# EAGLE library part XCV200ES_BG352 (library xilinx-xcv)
xcv200es_bg352 edit this description Auto generated by make-symbol-device-package-bsdl.ulp Rev. 26 Source: xcv200es_bg352.bsd
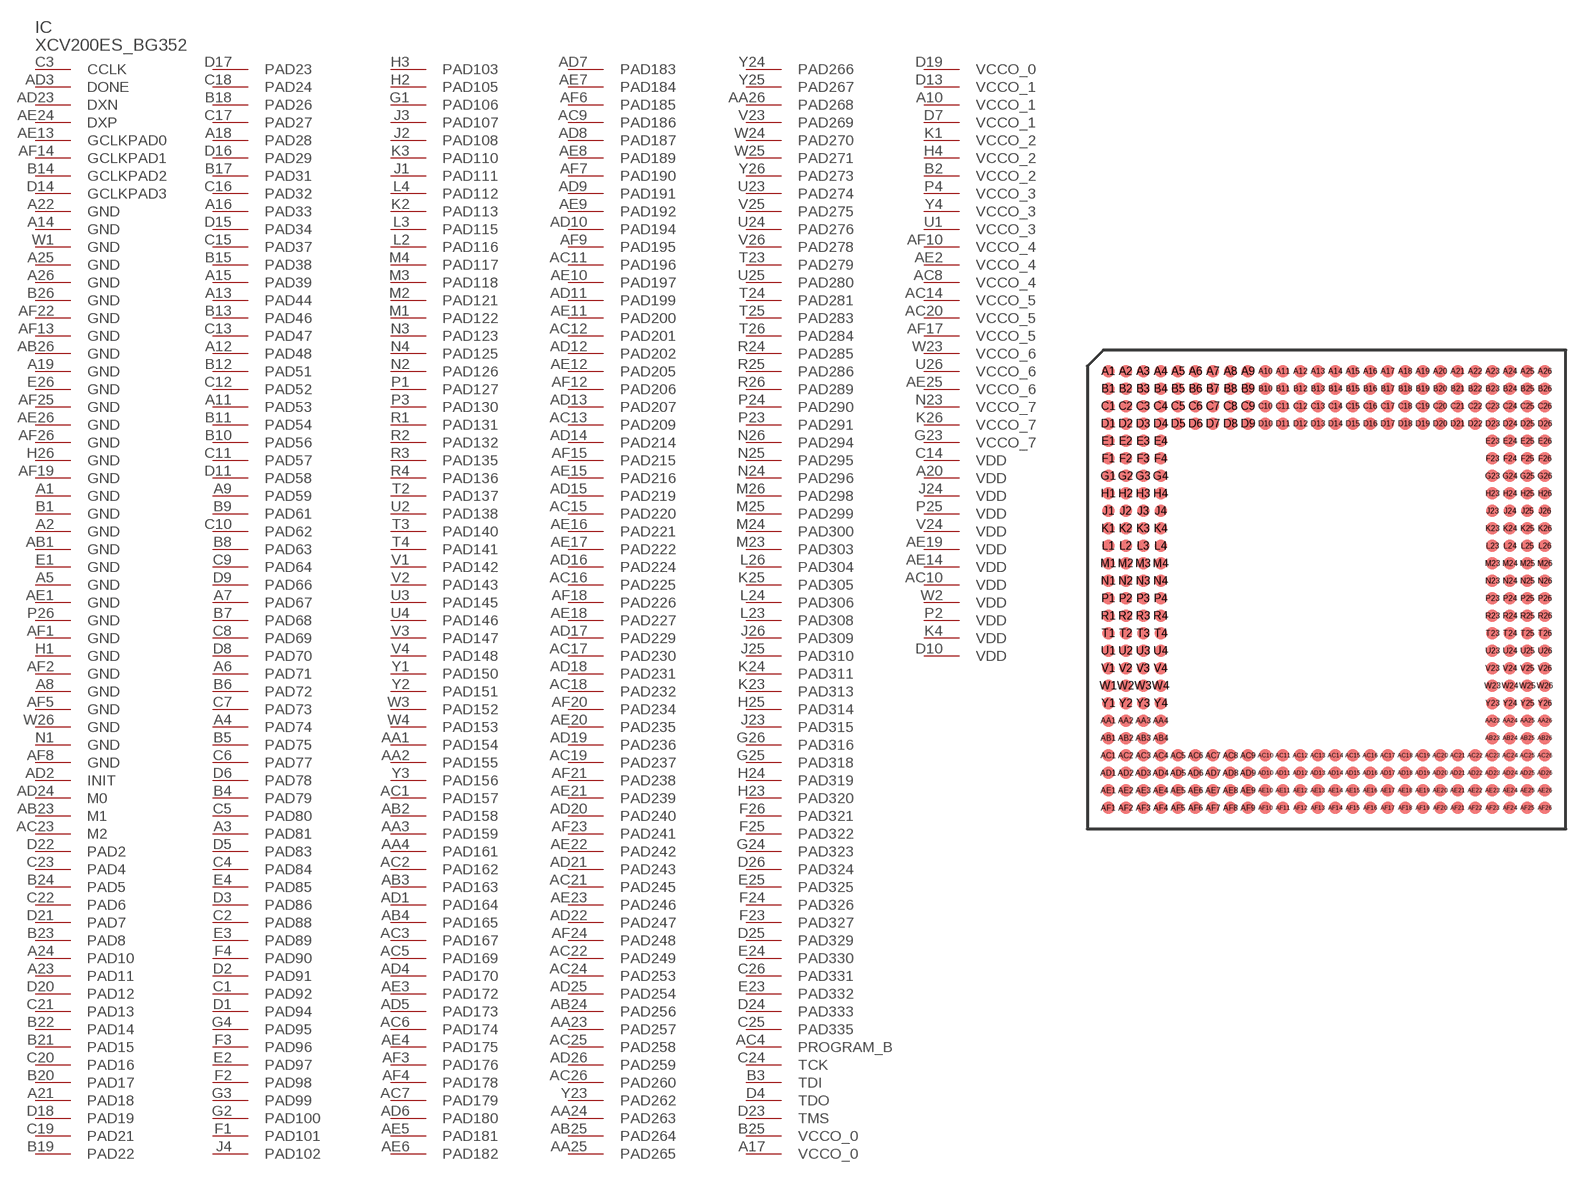
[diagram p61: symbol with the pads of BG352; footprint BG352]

Designator prefix IC

## XCV200ES_BG352 (OC_FARNELL: unknown; OC_NEWARK: unknown)  [BG352]
A1  GND  pwr
A2  GND  pwr
A3  PAD81
A4  PAD74
A5  GND  pwr
A6  PAD71
A7  PAD67
A8  GND  pwr
A9  PAD59
A10  VCCO_1  pwr
A11  PAD53
A12  PAD48
A13  PAD44
A14  GND  pwr
A15  PAD39
A16  PAD33
A17  VCCO_0  pwr
A18  PAD28
A19  GND  pwr
A20  VDD  pwr
A21  PAD18
A22  GND  pwr
A23  PAD11
A24  PAD10
A25  GND  pwr
A26  GND  pwr
AA1  PAD154
AA2  PAD155
AA3  PAD159
AA4  PAD161
AA23  PAD257
AA24  PAD263
AA25  PAD265
AA26  PAD268
AB1  GND  pwr
AB2  PAD158
AB3  PAD163
AB4  PAD165
AB23  M1  in
AB24  PAD256
AB25  PAD264
AB26  GND  pwr
AC1  PAD157
AC2  PAD162
AC3  PAD167
AC4  PROGRAM_B  in
AC5  PAD169
AC6  PAD174
AC7  PAD179
AC8  VCCO_4  pwr
AC9  PAD186
AC10  VDD  pwr
AC11  PAD196
AC12  PAD201
AC13  PAD209
AC14  VCCO_5  pwr
AC15  PAD220
AC16  PAD225
AC17  PAD230
AC18  PAD232
AC19  PAD237
AC20  VCCO_5  pwr
AC21  PAD245
AC22  PAD249
AC23  M2  in
AC24  PAD253
AC25  PAD258
AC26  PAD260
AD1  PAD164
AD2  INIT
AD3  DONE
AD4  PAD170
AD5  PAD173
AD6  PAD180
AD7  PAD183
AD8  PAD187
AD9  PAD191
AD10  PAD194
AD11  PAD199
AD12  PAD202
AD13  PAD207
AD14  PAD214
AD15  PAD219
AD16  PAD224
AD17  PAD229
AD18  PAD231
AD19  PAD236
AD20  PAD240
AD21  PAD243
AD22  PAD247
AD23  DXN  pas
AD24  M0  in
AD25  PAD254
AD26  PAD259
AE1  GND  pwr
AE2  VCCO_4  pwr
AE3  PAD172
AE4  PAD175
AE5  PAD181
AE6  PAD182
AE7  PAD184
AE8  PAD189
AE9  PAD192
AE10  PAD197
AE11  PAD200
AE12  PAD205
AE13  GCLKPAD0  in
AE14  VDD  pwr
AE15  PAD216
AE16  PAD221
AE17  PAD222
AE18  PAD227
AE19  VDD  pwr
AE20  PAD235
AE21  PAD239
AE22  PAD242
AE23  PAD246
AE24  DXP  pas
AE25  VCCO_6  pwr
AE26  GND  pwr
AF1  GND  pwr
AF2  GND  pwr
AF3  PAD176
AF4  PAD178
AF5  GND  pwr
AF6  PAD185
AF7  PAD190
AF8  GND  pwr
AF9  PAD195
AF10  VCCO_4  pwr
AF12  PAD206
AF13  GND  pwr
AF14  GCLKPAD1  in
AF15  PAD215
AF17  VCCO_5  pwr
AF18  PAD226
AF19  GND  pwr
AF20  PAD234
AF21  PAD238
AF22  GND  pwr
AF23  PAD241
AF24  PAD248
AF25  GND  pwr
AF26  GND  pwr
B1  GND  pwr
B2  VCCO_2  pwr
B3  TDI  in
B4  PAD79
B5  PAD75
B6  PAD72
B7  PAD68
B8  PAD63
B9  PAD61
B10  PAD56
B11  PAD54
B12  PAD51
B13  PAD46
B14  GCLKPAD2  in
B15  PAD38
B17  PAD31
B18  PAD26
B19  PAD22
B20  PAD17
B21  PAD15
B22  PAD14
B23  PAD8
B24  PAD5
B25  VCCO_0  pwr
B26  GND  pwr
C1  PAD92
C2  PAD88
C3  CCLK
C4  PAD84
C5  PAD80
C6  PAD77
C7  PAD73
C8  PAD69
C9  PAD64
C10  PAD62
C11  PAD57
C12  PAD52
C13  PAD47
C14  VDD  pwr
C15  PAD37
C16  PAD32
C17  PAD27
C18  PAD24
C19  PAD21
C20  PAD16
C21  PAD13
C22  PAD6
C23  PAD4
C24  TCK  in
C25  PAD335
C26  PAD331
D1  PAD94
D2  PAD91
D3  PAD86
D4  TDO  out
D5  PAD83
D6  PAD78
D7  VCCO_1  pwr
D8  PAD70
D9  PAD66
D10  VDD  pwr
D11  PAD58
D13  VCCO_1  pwr
D14  GCLKPAD3  in
D15  PAD34
D16  PAD29
D17  PAD23
D18  PAD19
D19  VCCO_0  pwr
D20  PAD12
D21  PAD7
D22  PAD2
D23  TMS  in
D24  PAD333
D25  PAD329
D26  PAD324
E1  GND  pwr
E2  PAD97
E3  PAD89
E4  PAD85
E23  PAD332
E24  PAD330
E25  PAD325
E26  GND  pwr
F1  PAD101
F2  PAD98
F3  PAD96
F4  PAD90
F23  PAD327
F24  PAD326
F25  PAD322
F26  PAD321
G1  PAD106
G2  PAD100
G3  PAD99
G4  PAD95
G23  VCCO_7  pwr
G24  PAD323
G25  PAD318
G26  PAD316
H1  GND  pwr
H2  PAD105
H3  PAD103
H4  VCCO_2  pwr
H23  PAD320
H24  PAD319
H25  PAD314
H26  GND  pwr
J1  PAD111
J2  PAD108
J3  PAD107
J4  PAD102
J23  PAD315
J24  VDD  pwr
J25  PAD310
J26  PAD309
K1  VCCO_2  pwr
K2  PAD113
K3  PAD110
K4  VDD  pwr
K23  PAD313
K24  PAD311
K25  PAD305
K26  VCCO_7  pwr
L2  PAD116
L3  PAD115
L4  PAD112
L23  PAD308
L24  PAD306
L26  PAD304
M1  PAD122
M2  PAD121
M3  PAD118
M4  PAD117
M23  PAD303
M24  PAD300
M25  PAD299
M26  PAD298
N1  GND  pwr
N2  PAD126
N3  PAD123
N4  PAD125
N23  VCCO_7  pwr
N24  PAD296
N25  PAD295
N26  PAD294
P1  PAD127
P2  VDD  pwr
P3  PAD130
P4  VCCO_3  pwr
P23  PAD291
P24  PAD290
P25  VDD  pwr
P26  GND  pwr
R1  PAD131
R2  PAD132
R3  PAD135
R4  PAD136
R24  PAD285
R25  PAD286
R26  PAD289
T2  PAD137
T3  PAD140
T4  PAD141
T23  PAD279
T24  PAD281
T25  PAD283
T26  PAD284
U1  VCCO_3  pwr
U2  PAD138
U3  PAD145
U4  PAD146
U23  PAD274
U24  PAD276
U25  PAD280
U26  VCCO_6  pwr
V1  PAD142
V2  PAD143
V3  PAD147
V4  PAD148
V23  PAD269
V24  VDD  pwr
V25  PAD275
V26  PAD278
W1  GND  pwr
W2  VDD  pwr
W3  PAD152
W4  PAD153
W23  VCCO_6  pwr
W24  PAD270
W25  PAD271
W26  GND  pwr
Y1  PAD150
Y2  PAD151
Y3  PAD156
Y4  VCCO_3  pwr
Y23  PAD262
Y24  PAD266
Y25  PAD267
Y26  PAD273

## Footprint BG352 (pad centres in mm)
xcv100e_bg352 edit this description Auto generated by make-symbol-device-package-bsdl.ulp Rev. 26 Source: xcv100e_bg352.bsd
smd 0.9 x 0.9: A1 -15.875,15.875; A2 -14.605,15.875; A3 -13.335,15.875; A4 -12.065,15.875; A5 -10.795,15.875; A6 -9.525,15.875; A7 -8.255,15.875; A8 -6.985,15.875; A9 -5.715,15.875; A10 -4.445,15.875; A11 -3.175,15.875; A12 -1.905,15.875; A13 -0.635,15.875; A14 0.635,15.875; A15 1.905,15.875; A16 3.175,15.875; A17 4.445,15.875; A18 5.715,15.875; A19 6.985,15.875; A20 8.255,15.875; A21 9.525,15.875; A22 10.795,15.875; A23 12.065,15.875; A24 13.335,15.875; A25 14.605,15.875; A26 15.875,15.875; AA1 -15.875,-9.525; AA2 -14.605,-9.525; AA3 -13.335,-9.525; AA4 -12.065,-9.525; AA23 12.065,-9.525; AA24 13.335,-9.525; AA25 14.605,-9.525; AA26 15.875,-9.525; AB1 -15.875,-10.795; AB2 -14.605,-10.795; AB3 -13.335,-10.795; AB4 -12.065,-10.795; AB23 12.065,-10.795; AB24 13.335,-10.795; AB25 14.605,-10.795; AB26 15.875,-10.795; AC1 -15.875,-12.065; AC2 -14.605,-12.065; AC3 -13.335,-12.065; AC4 -12.065,-12.065; AC5 -10.795,-12.065; AC6 -9.525,-12.065; AC7 -8.255,-12.065; AC8 -6.985,-12.065; AC9 -5.715,-12.065; AC10 -4.445,-12.065; AC11 -3.175,-12.065; AC12 -1.905,-12.065; AC13 -0.635,-12.065; AC14 0.635,-12.065; AC15 1.905,-12.065; AC16 3.175,-12.065; AC17 4.445,-12.065; AC18 5.715,-12.065; AC19 6.985,-12.065; AC20 8.255,-12.065; AC21 9.525,-12.065; AC22 10.795,-12.065; AC23 12.065,-12.065; AC24 13.335,-12.065; AC25 14.605,-12.065; AC26 15.875,-12.065; AD1 -15.875,-13.335; AD2 -14.605,-13.335; AD3 -13.335,-13.335; AD4 -12.065,-13.335; AD5 -10.795,-13.335; AD6 -9.525,-13.335; AD7 -8.255,-13.335; AD8 -6.985,-13.335; AD9 -5.715,-13.335; AD10 -4.445,-13.335; AD11 -3.175,-13.335; AD12 -1.905,-13.335; AD13 -0.635,-13.335; AD14 0.635,-13.335; AD15 1.905,-13.335; AD16 3.175,-13.335; AD17 4.445,-13.335; AD18 5.715,-13.335; AD19 6.985,-13.335; AD20 8.255,-13.335; AD21 9.525,-13.335; AD22 10.795,-13.335; AD23 12.065,-13.335; AD24 13.335,-13.335; AD25 14.605,-13.335; AD26 15.875,-13.335; AE1 -15.875,-14.605; AE2 -14.605,-14.605; AE3 -13.335,-14.605; AE4 -12.065,-14.605; AE5 -10.795,-14.605; AE6 -9.525,-14.605; AE7 -8.255,-14.605; AE8 -6.985,-14.605; AE9 -5.715,-14.605; AE10 -4.445,-14.605; AE11 -3.175,-14.605; AE12 -1.905,-14.605; AE13 -0.635,-14.605; AE14 0.635,-14.605; AE15 1.905,-14.605; AE16 3.175,-14.605; AE17 4.445,-14.605; AE18 5.715,-14.605; AE19 6.985,-14.605; AE20 8.255,-14.605; AE21 9.525,-14.605; AE22 10.795,-14.605; AE23 12.065,-14.605; AE24 13.335,-14.605; AE25 14.605,-14.605; AE26 15.875,-14.605; AF1 -15.875,-15.875; AF2 -14.605,-15.875; AF3 -13.335,-15.875; AF4 -12.065,-15.875; AF5 -10.795,-15.875; AF6 -9.525,-15.875; AF7 -8.255,-15.875; AF8 -6.985,-15.875; AF9 -5.715,-15.875; AF10 -4.445,-15.875; AF11 -3.175,-15.875; AF12 -1.905,-15.875; AF13 -0.635,-15.875; AF14 0.635,-15.875; AF15 1.905,-15.875; AF16 3.175,-15.875; AF17 4.445,-15.875; AF18 5.715,-15.875; AF19 6.985,-15.875; AF20 8.255,-15.875; AF21 9.525,-15.875; AF22 10.795,-15.875; AF23 12.065,-15.875; AF24 13.335,-15.875; AF25 14.605,-15.875; AF26 15.875,-15.875; B1 -15.875,14.605; B2 -14.605,14.605; B3 -13.335,14.605; B4 -12.065,14.605; B5 -10.795,14.605; B6 -9.525,14.605; B7 -8.255,14.605; B8 -6.985,14.605; B9 -5.715,14.605; B10 -4.445,14.605; B11 -3.175,14.605; B12 -1.905,14.605; B13 -0.635,14.605; B14 0.635,14.605; B15 1.905,14.605; B16 3.175,14.605; B17 4.445,14.605; B18 5.715,14.605; B19 6.985,14.605; B20 8.255,14.605; B21 9.525,14.605; B22 10.795,14.605; B23 12.065,14.605; B24 13.335,14.605; B25 14.605,14.605; B26 15.875,14.605; C1 -15.875,13.335; C2 -14.605,13.335; C3 -13.335,13.335; C4 -12.065,13.335; C5 -10.795,13.335; C6 -9.525,13.335; C7 -8.255,13.335; C8 -6.985,13.335; C9 -5.715,13.335; C10 -4.445,13.335; C11 -3.175,13.335; C12 -1.905,13.335; C13 -0.635,13.335; C14 0.635,13.335; C15 1.905,13.335; C16 3.175,13.335; C17 4.445,13.335; C18 5.715,13.335; C19 6.985,13.335; C20 8.255,13.335; C21 9.525,13.335; C22 10.795,13.335; C23 12.065,13.335; C24 13.335,13.335; C25 14.605,13.335; C26 15.875,13.335; D1 -15.875,12.065; D2 -14.605,12.065; D3 -13.335,12.065; D4 -12.065,12.065; D5 -10.795,12.065; D6 -9.525,12.065; D7 -8.255,12.065; D8 -6.985,12.065; D9 -5.715,12.065; D10 -4.445,12.065; D11 -3.175,12.065; D12 -1.905,12.065; D13 -0.635,12.065; D14 0.635,12.065; D15 1.905,12.065; D16 3.175,12.065; D17 4.445,12.065; D18 5.715,12.065; D19 6.985,12.065; D20 8.255,12.065; D21 9.525,12.065; D22 10.795,12.065; D23 12.065,12.065; D24 13.335,12.065; D25 14.605,12.065; D26 15.875,12.065; E1 -15.875,10.795; E2 -14.605,10.795; E3 -13.335,10.795; E4 -12.065,10.795; E23 12.065,10.795; E24 13.335,10.795; E25 14.605,10.795; E26 15.875,10.795; F1 -15.875,9.525; F2 -14.605,9.525; F3 -13.335,9.525; F4 -12.065,9.525; F23 12.065,9.525; F24 13.335,9.525; F25 14.605,9.525; F26 15.875,9.525; G1 -15.875,8.255; G2 -14.605,8.255; G3 -13.335,8.255; G4 -12.065,8.255; G23 12.065,8.255; G24 13.335,8.255; G25 14.605,8.255; G26 15.875,8.255; H1 -15.875,6.985; H2 -14.605,6.985; H3 -13.335,6.985; H4 -12.065,6.985; H23 12.065,6.985; H24 13.335,6.985; H25 14.605,6.985; H26 15.875,6.985; J1 -15.875,5.715; J2 -14.605,5.715; J3 -13.335,5.715; J4 -12.065,5.715; J23 12.065,5.715; J24 13.335,5.715; J25 14.605,5.715; J26 15.875,5.715; K1 -15.875,4.445; K2 -14.605,4.445; K3 -13.335,4.445; K4 -12.065,4.445; K23 12.065,4.445; K24 13.335,4.445; K25 14.605,4.445; K26 15.875,4.445; L1 -15.875,3.175; L2 -14.605,3.175; L3 -13.335,3.175; L4 -12.065,3.175; L23 12.065,3.175; L24 13.335,3.175; L25 14.605,3.175; L26 15.875,3.175; M1 -15.875,1.905; M2 -14.605,1.905; M3 -13.335,1.905; M4 -12.065,1.905; M23 12.065,1.905; M24 13.335,1.905; M25 14.605,1.905; M26 15.875,1.905; N1 -15.875,0.635; N2 -14.605,0.635; N3 -13.335,0.635; N4 -12.065,0.635; N23 12.065,0.635; N24 13.335,0.635; N25 14.605,0.635; N26 15.875,0.635; P1 -15.875,-0.635; P2 -14.605,-0.635; P3 -13.335,-0.635; P4 -12.065,-0.635; P23 12.065,-0.635; P24 13.335,-0.635; P25 14.605,-0.635; P26 15.875,-0.635; R1 -15.875,-1.905; R2 -14.605,-1.905; R3 -13.335,-1.905; R4 -12.065,-1.905; R23 12.065,-1.905; R24 13.335,-1.905; R25 14.605,-1.905; R26 15.875,-1.905; T1 -15.875,-3.175; T2 -14.605,-3.175; T3 -13.335,-3.175; T4 -12.065,-3.175; T23 12.065,-3.175; T24 13.335,-3.175; T25 14.605,-3.175; T26 15.875,-3.175; U1 -15.875,-4.445; U2 -14.605,-4.445; U3 -13.335,-4.445; U4 -12.065,-4.445; U23 12.065,-4.445; U24 13.335,-4.445; U25 14.605,-4.445; U26 15.875,-4.445; V1 -15.875,-5.715; V2 -14.605,-5.715; V3 -13.335,-5.715; V4 -12.065,-5.715; V23 12.065,-5.715; V24 13.335,-5.715; V25 14.605,-5.715; V26 15.875,-5.715; W1 -15.875,-6.985; W2 -14.605,-6.985; W3 -13.335,-6.985; W4 -12.065,-6.985; W23 12.065,-6.985; W24 13.335,-6.985; W25 14.605,-6.985; W26 15.875,-6.985; Y1 -15.875,-8.255; Y2 -14.605,-8.255; Y3 -13.335,-8.255; Y4 -12.065,-8.255; Y23 12.065,-8.255; Y24 13.335,-8.255; Y25 14.605,-8.255; Y26 15.875,-8.255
